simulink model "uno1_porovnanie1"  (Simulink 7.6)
settings: Solver=ode4  StartTime=0.0  StopTime=50  FixedStep=0.2  RelTol=1e-3
undefined symbols (not defined in the file or in its folder): ABOVE_NORMAL_PRIORITY, COM3, lightbulb

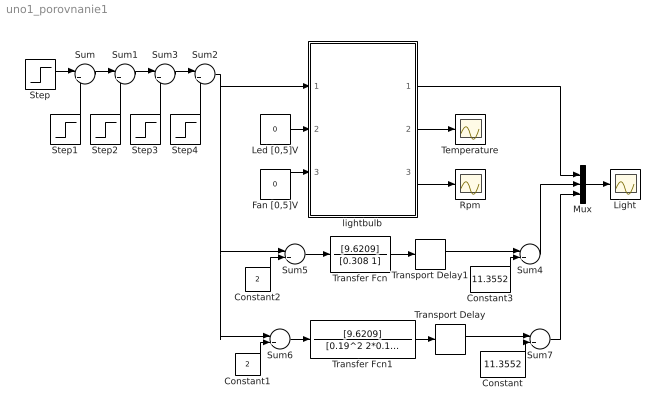
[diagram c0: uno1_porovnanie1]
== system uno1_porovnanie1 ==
  Constant : Constant  Value=11.3552
  Constant1 : Constant  Value=2
  Constant2 : Constant  Value=2
  Constant3 : Constant  Value=11.3552
  Fan [0,5]V : Constant  Value=0
  Led [0,5]V : Constant  Value=0
  Light : Scope
  Mux : Mux  Inputs=3
  Rpm : Scope
  Step : Step  Time=0  After=2  SampleTime=0
  Step1 : Step  Time=10  After=3  SampleTime=0
  Step2 : Step  Time=20  After=-2  SampleTime=0
  Step3 : Step  Time=30  After=-2  SampleTime=0
  Step4 : Step  Time=40  After=3  SampleTime=0
  Sum{,1..4,7} (6 alike) : Sum  Inputs=|++
  Sum5 : Sum  Inputs=|+-
  Sum6 : Sum  Inputs=|+-
  Temperature : Scope
  Transfer Fcn : TransferFcn  Numerator=[9.6209]  Denominator=[0.308 1]
  Transfer Fcn1 : TransferFcn  Numerator=[9.6209]  Denominator=[0.19^2 2*0.19 1]
  Transport Delay : TransportDelay  DelayTime=0.4
  Transport Delay1 : TransportDelay  DelayTime=0.515
  lightbulb : Subsystem  AncestorBlock=lightbulb/lightbulb
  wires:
  Fan [0,5]V/1 -> lightbulb/3(fan)
  lightbulb/2(temperature) -> Temperature/1
  lightbulb/3(rpm) -> Rpm/1
  Led [0,5]V/1 -> lightbulb/2(led)
  Step/1 -> Sum/1
  Step2/1 -> Sum1/2
  Step3/1 -> Sum3/2
  Step4/1 -> Sum2/2
  Sum/1 -> Sum1/1
  Sum1/1 -> Sum3/1
  Sum3/1 -> Sum2/1
  Sum2/1 -> lightbulb/1(bulb), Sum5/1, Sum6/1
  lightbulb/1(light) -> Mux/1
  Mux/1 -> Light/1
  Transfer Fcn/1 -> Transport Delay1/1
  Transfer Fcn1/1 -> Transport Delay/1
  Sum5/1 -> Transfer Fcn/1
  Sum6/1 -> Transfer Fcn1/1
  Transport Delay/1 -> Sum7/1
  Transport Delay1/1 -> Sum4/1
  Constant2/1 -> Sum5/2
  Constant1/1 -> Sum6/2
  Constant3/1 -> Sum4/2
  Constant/1 -> Sum7/2
  Step1/1 -> Sum/2
  Sum7/1 -> Mux/3
  Sum4/1 -> Mux/2

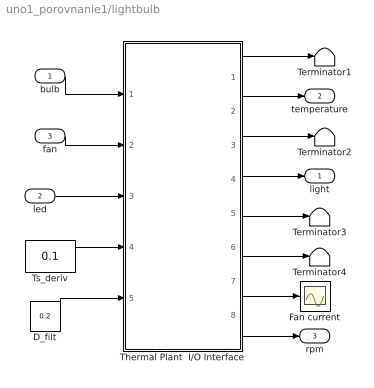
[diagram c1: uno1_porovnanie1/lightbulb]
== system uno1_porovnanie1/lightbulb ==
  bulb : Inport
  led : Inport  Port=2
  fan : Inport  Port=3
  D_filt : Constant  Value=0.2
  Fan current : Scope
  Terminator{1..4} (4 alike) : Terminator
  Thermal Plant  I/O Interface : Subsystem  mask{Ts=0.2}
      mask prompts: Ts "Sample time (s)"
      mask init:
      | set_param(bdroot,'FixedStep',num2str(Ts));
  Ts_deriv : Constant  Value=0.1
  light : Outport
  temperature : Outport  Port=2
  rpm : Outport  Port=3
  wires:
  bulb/1 -> Thermal Plant  I/O Interface/1(Bulb)
  Thermal Plant  I/O Interface/8(Fan rpm) -> rpm/1
  Thermal Plant  I/O Interface/7(Fan current) -> Fan current/1
  D_filt/1 -> Thermal Plant  I/O Interface/5(D_filt)
  Ts_deriv/1 -> Thermal Plant  I/O Interface/4(Ts_deriv)
  led/1 -> Thermal Plant  I/O Interface/3(LED)
  fan/1 -> Thermal Plant  I/O Interface/2(Fan)
  Thermal Plant  I/O Interface/1(Ambient temperature) -> Terminator1/1
  Thermal Plant  I/O Interface/6(Derivative  of light intensity) -> Terminator4/1
  Thermal Plant  I/O Interface/5(Filtered light intensity) -> Terminator3/1
  Thermal Plant  I/O Interface/4(Light intensity) -> light/1
  Thermal Plant  I/O Interface/2(Temperature) -> temperature/1
  Thermal Plant  I/O Interface/3(Filtered temperature) -> Terminator2/1

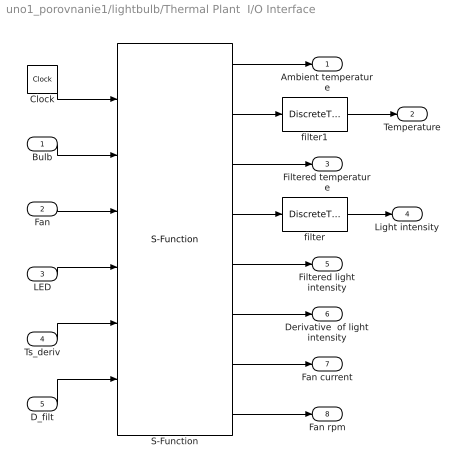
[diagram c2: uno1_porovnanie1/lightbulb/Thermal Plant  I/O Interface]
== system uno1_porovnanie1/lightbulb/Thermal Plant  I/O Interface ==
  Bulb : Inport
  Fan : Inport  Port=2
  LED : Inport  Port=3
  Ts_deriv : Inport  Port=4
  D_filt : Inport  Port=5
  Clock : Clock
  S-Function : S-Function  Priority=1  FunctionName=udaq28LT_v1R13  Parameters=com_port, Ts, events_ot, rd_timeout, matlab_prior, warning, printout  EnableBusSupport=off  mask(uDAQ28/LT Communication Interface){com_port=COM3, Ts=Ts, events_ot=1, rd_timeout=Ts/2*1000, matlab_prior=ABOVE_NORMAL_PRIORITY, warning=on, printout=off}
      mask prompts: com_port "Serial port:"; Ts "Sample time (sec):"; events_ot "Sampling delayed (%):"; rd_timeout "Read timeout (msec, lower than sample time):"; matlab_prior "Matlab priority"; warning "Warning if delayed (error if unchecked)"; printout "Detailed timing and timeout  printout"
      mask help: (c) 2006 Martin Kamensky Serial port - USB serial port number assigned to uDAQ28/LT system Sampling time (sec) - the lowest working value in Windows is about 0.04 - 0.05 s Sample delayed (%) - number of events (percentually) when simulink loop can take more than time determined by sample time Read timeout (msec) - timeout for reading data from the port (the lowest working value is about 25 ms) Matlab priority : NORMAL_PRIORITY - priority of common Windows application ABOVE_NORMAL_PRIORITY - recommended - higher priority than common Windows application priority HIGH_PRIORITY - recommended - hig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
      mask init:
      | %set_param(bdroot,'FixedStep',get_param(gcb,'Ts'));
      | set_param(bdroot,'Solver','ode4');
  filter : DiscreteTransferFcn  Numerator=0.6  Denominator=[1 -0.4]  SampleTime=Ts
  filter1 : DiscreteTransferFcn  Numerator=0.6  Denominator=[1 -0.4]  SampleTime=Ts
  Ambient temperature : Outport
  Temperature : Outport  Port=2
  Filtered temperature : Outport  Port=3
  Light intensity : Outport  Port=4
  Filtered light intensity : Outport  Port=5
  Derivative  of light intensity : Outport  Port=6
  Fan current : Outport  Port=7
  Fan rpm : Outport  Port=8
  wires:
  S-Function/8 -> Fan rpm/1
  S-Function/7 -> Fan current/1
  S-Function/6 -> Derivative  of light intensity/1
  S-Function/5 -> Filtered light intensity/1
  S-Function/4 -> filter/1
  S-Function/3 -> Filtered temperature/1
  S-Function/2 -> filter1/1
  S-Function/1 -> Ambient temperature/1
  D_filt/1 -> S-Function/6
  Ts_deriv/1 -> S-Function/5
  LED/1 -> S-Function/4
  Fan/1 -> S-Function/3
  Bulb/1 -> S-Function/2
  Clock/1 -> S-Function/1
  filter1/1 -> Temperature/1
  filter/1 -> Light intensity/1
